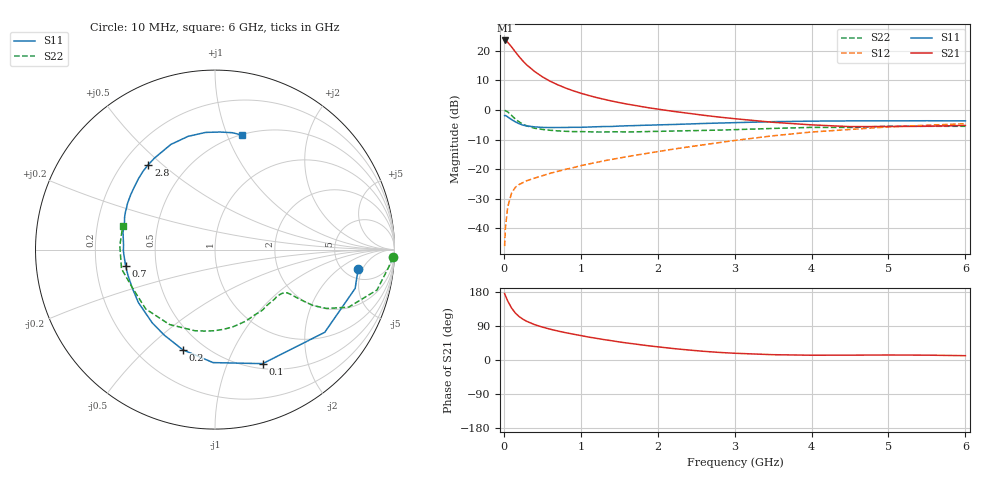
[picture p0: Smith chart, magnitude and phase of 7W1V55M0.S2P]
! Infineon Technologies  Discrete & RF Semiconductors
! BFS17W
! Si NPN RF Bipolar Junction Transistor in SOT323
! VCE = 1.5 V  IC = 5 mA
! Common Emitter S-Parameters:  August  1999
# GHz  S  MA  R  50
!  f  S11  S21  S12  S22
! GHz  MAG  ANG  MAG  ANG  MAG  ANG  MAG  ANG
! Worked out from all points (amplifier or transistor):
!   36 points, 10 MHz to 6 GHz, reference 50 ohm
!   highest |S21| = 23.5 dB at 20 MHz (marker M1)
!   |S21| within 3 dB of that: start of sweep to 124.4 MHz
!   unconditionally stable (mu >= 1): 523.9 MHz to end of sweep
!   at 250 MHz: K = 0.61, MSG = 20.5 dB, |S12| = -24.5 dB
!   at 1.4 GHz: K = 1.30, MAG = 6.6 dB, |S12| = -16.7 dB
!   at 6 GHz: K = 1.11, MAG = -2.3 dB, |S12| = -4.6 dB
!   S11 on the Smith chart (normalised r, x): 10 MHz: 6.75, -4.09; 100 MHz: 0.56, -1.35; 200 MHz: 0.39, -0.66; 700 MHz: 0.33, -0.08; 2.8 GHz: 0.30, +0.45; 6 GHz: 0.51, +1.13
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0.01  0.8052 -7.6  14.95 175.6  0.005 84.1  0.9911 -2.5
0.02  0.8102 -15.5  14.98 170.0  0.01 87.8  0.9718 -5.9
0.05  0.7656 -37.0  13.96 155.9  0.0229 72.4  0.9301 -14.0
0.1  0.6887 -67.3  11.68 137.4  0.0393 59.5  0.8106 -23.3
0.15  0.6297 -91.0  9.582 123.8  0.0495 51.6  0.7035 -27.8
0.2  0.5863 -107.8  7.951 114.4  0.0553 47.8  0.6283 -29.7
0.25  0.5542 -120.6  6.69 107.4  0.0595 45.5  0.5726 -30.2
0.3  0.5374 -130.6  5.754 101.9  0.064 45.6  0.539 -30.4
0.4  0.5189 -145.4  4.474 93.3  0.0706 45.7  0.4922 -30.6
0.5  0.5081 -155.5  3.648 86.9  0.0775 47.5  0.4699 -30.9
0.6  0.5055 -163.3  3.073 81.4  0.085 49.3  0.4548 -31.9
0.7  0.5063 -169.4  2.672 76.6  0.092 50.9  0.4442 -33.5
0.9  0.5106 -179.2  2.116 68.3  0.106 53.9  0.4319 -37.5
1.1  0.5152 172.8  1.765 60.6  0.1224 55.9  0.4287 -42.5
1.3  0.5256 165.7  1.519 53.9  0.1384 57.1  0.4244 -48.3
1.6  0.5414 157.1  1.26 44.9  0.1623 58.5  0.4258 -57.2
2.2  0.5691 142.2  0.95 30.3  0.218 59.6  0.4417 -76.9
2.8  0.6019 128.1  0.759 20.0  0.2815 57.9  0.4577 -97.5
3.5  0.6354 112.8  0.62 14.0  0.3669 52.9  0.4884 -121.3
4.5  0.655 94.6  0.524 12.8  0.4691 41.1  0.5068 -155.1
5.5  0.6585 81.5  0.531 12.8  0.5531 29.5  0.5308 177.7
6  0.6554 76.6  0.549 11.4  0.5864 24.0  0.5305 165.7
